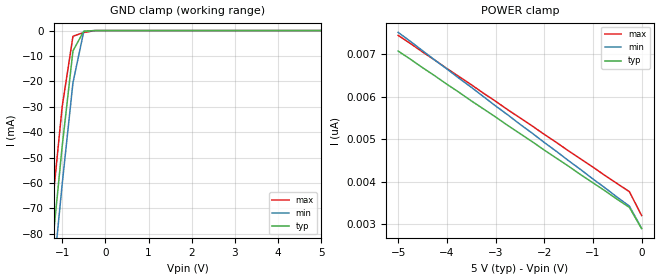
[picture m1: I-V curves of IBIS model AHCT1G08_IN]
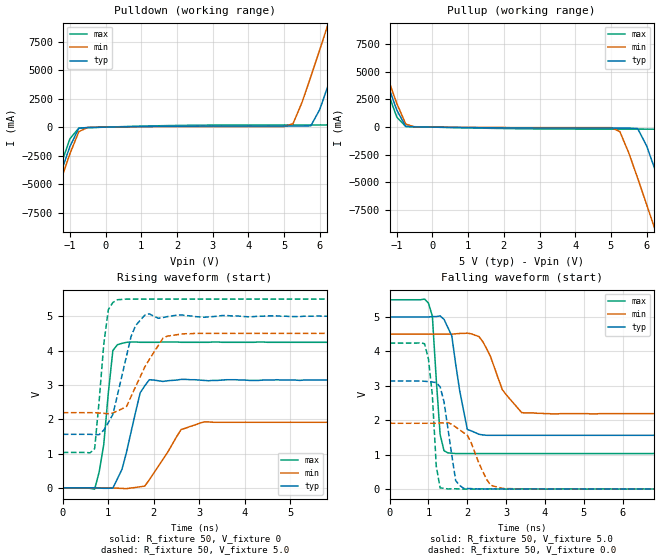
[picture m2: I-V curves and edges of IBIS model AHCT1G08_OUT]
| TEXAS INSTRUMENTS INCORPORATED
| Standard Linear and Logic Group
| IBIS Model of SN74AHCT1G08
| SINGLE 2-INPUT POSITIVE-AND GATE
| SOT 5-pin (DCK) and SOT 5-pin (DBV) Package
[IBIS Ver]   3.2
[Comment Char]  |_char
[File Name]   ahct1g08.ibs
[File Rev]   2.0 J_die
[Date]   May 24, 2000
[Source]   Data created from HSPICE simulations at TI-SLL.
[Notes]   The following is an IBIS list for the AHCT1G08.
|   Please contact sllibis@ti.com with questions and
|   comments concerning SLL IBIS models.
[Disclaimer] Property of Texas Instruments Incorporated.  Unauthorized
   reproduction and/or distribution is strictly prohibited.
   This product is protected under copyright law.
   Created 2000, (C) Copyright 2000, Texas Instruments Inc.,
   All Rights Reserved.
   UNLESS THERE IS A SIGNED, WRITTEN AGREEMENT TO THE
   CONTRARY, TEXAS INSTRUMENTS () IS PROVIDING THE IBIS
   MODELS  AND WITHOUT ANY WARRANTY, EXPRESSED OR
   IMPLIED.  TI assumes no liability for:
   1) the accuracy of the IBIS models provided to your
   company;
   2) the proper functioning of these IBIS Models in your
   design or for any resulting applications; or
   3) infringement of patents, copyrights or intellectual
   property rights resulting from your use of these IBIS
   models.
   TI provides IBIS Models as a service to our customers.
   You and your company shall not distribute, sell or give
   these models to anyone else without prior written
   permission from TI.
   TI reserves the right to make changes to our products or
   to discontinue any semiconductor product or service
   without notice, and advises our customers to obtain the
   latest version of relevant information to verify, before
   placing orders, that the information being relied on is
   current.
   Please be aware that your receipt and use of the IBIS
   information provided shall serve as acceptance of these
   terms and conditions.  If you do not accept these terms,
   you should return or destroy the IBIS models and any
   other accompanying information immediately.
|   Component AHCT1G08_DCK
[Component]   AHCT1G08_DCK
[Manufacturer]  Texas Instruments, Inc.
[Package]
|   typ   min   max
R_pkg   0.020   0.017   0.025
L_pkg   0.998nH   0.881nH   1.069nH
C_pkg   0.146pF   0.118pF   0.205pF
[Pin]   signal_name   model_name   R_pin   L_pin   C_pin
1   A   AHCT1G08_IN   0.019   1.069nH   0.162pF
2   B   AHCT1G08_IN   0.018   0.881nH   0.121pF
3   GND   GND   0.017   1.031nH   0.205pF
4   Y   AHCT1G08_OUT   0.020   0.960nH   0.124pF
5   VCC   POWER   0.025   1.049nH   0.118pF
|   Component AHCT1G08_DBV
[Component]   AHCT1G08_DBV
[Manufacturer]  Texas Instruments, Inc.
[Package]
|   typ   min   max
R_pkg   0.025   0.021   0.029
L_pkg   1.529nH   1.312nH   1.906nH
C_pkg   0.156pF   0.110pF   0.240pF
[Pin]   signal_name   model_name   R_pin   L_pin   C_pin
1   A   AHCT1G08_IN   0.021   1.511nH   0.144pF
2   B   AHCT1G08_IN   0.023   1.312nH   0.138pF
3   GND   GND   0.029   1.906nH   0.240pF
4   Y   AHCT1G08_OUT   0.026   1.541nH   0.150pF
5   VCC   POWER   0.025   1.374nH   0.110pF
| Models and submodels in the file (2): AHCT1G08_IN (Input), AHCT1G08_OUT (Output)
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|   Model AHCT1G08_IN
[Model]   AHCT1G08_IN
Model_type  Input
Polarity   Inverting
Vinl = 0.8
Vinh = 2.0
| variable   typ   min   max
C_comp   1.24pf   0.93pf   1.55pf
[Temperature Range]   25   85   -40
[Voltage Range]   5.0   4.5   5.5
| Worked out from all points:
|   GND clamp passes 1 mA (typ) near -0.52 V on its own axis
[GND Clamp]
|   Voltage   I(typ)   I(min)   I(max)
-5V       -773mA     -786mA     -758mA
-1.5V     -133mA     -148mA     -117mA
-1.25V    -88.7mA    -104mA     -72.7mA
-1V       -45.6mA    -60.5mA    -30mA
-750mV    -7.99mA    -20.5mA    -2.23mA
-500mV    -233uA     -353uA     -759uA
-250mV    -2.63nA    -182nA     -26.9uA
5V        2.9nA      3.64nA     2.54nA
[POWER Clamp]
|   Voltage   I(typ)   I(min)   I(max)
-5V       7.08nA     7.52nA     7.45nA
-1.5V     4.37nA     4.5nA      4.73nA
-250mV    3.4nA      3.43nA     3.77nA
0V        2.9nA      2.91nA     3.21nA
|   Model AHCT1G08_OUT
[Model]   AHCT1G08_OUT
Model_type  Output
Polarity   Inverting
Vmeas = 2.50v
Cref = 15pf
| variable   typ   min   max
C_comp   3.12pf   2.34pf   3.90pf
[Temperature Range]   25   85   -40
[Voltage Range]   5.0   4.5   5.5
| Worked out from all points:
|   slope of the pulldown table from 0 to 0.75 V, typ, clamps not added: 18.8 ohm
|   slope of the pullup table from 0 to 0.75 V, typ, clamps not added: 25.3 ohm
|   rising waveform, R_fixture 50, V_fixture 0: 20-80 % time 336ps typ, 543ps min, 203ps max; typ from 0 V to 3.14 V
|   falling waveform, R_fixture 50, V_fixture 5.0: 20-80 % time 292ps typ, 554ps min, 156ps max; typ from 5 V to 1.56 V
|   rising waveform, R_fixture 50, V_fixture 5.0: 20-80 % time 364ps typ, 547ps min, 187ps max; typ from 1.56 V to 5 V
|   falling waveform, R_fixture 50, V_fixture 0.0: 20-80 % time 246ps typ, 438ps min, 155ps max; typ from 3.14 V to 0 V
[Pulldown]
|   Voltage   I(typ)   I(min)   I(max)
-5V       -40.9A     -41.4A     -40.3A
-1.75V    -8.76A     -9.39A     -8.09A
-1V       -1.69A     -2.33A     -1.02A
-750mV    -95.5mA    -395mA     -80.6mA
5.25V     93.4mA     298mA      192mA
5.75V     116mA      4.42A      192mA
6.25V     3.8A       9.19A      193mA
6.5V      6.17A      11.6A      931mA
6.75V     8.59A      14.1A      3.15A
7.25V     13.5A      19A        7.96A
7.5V      15.9A      21.4A      10.4A
10V       40.7A      46.2A      35.2A
[Pullup]
|   Voltage   I(typ)   I(min)   I(max)
-5V       40.7A      41.2A      40.1A
-2V       11A        11.6A      10.4A
-1.75V    8.59A      9.19A      7.96A
-1V       1.54A      2.14A      907mA
-750mV    63.6mA     284mA      62.5mA
5.25V     -84.4mA    -401mA     -178mA
5.75V     -130mA     -4.62A     -178mA
6.25V     -3.97A     -9.39A     -187mA
6.75V     -8.76A     -14.3A     -3.28A
7.25V     -13.6A     -19.2A     -8.09A
7.5V      -16.1A     -21.6A     -10.5A
10V       -40.9A     -46.4A     -35.3A
[Ramp]
| variable   typ   min   max
dV/dt_r   1.89E+00/3.19E-10   1.16E+00/5.23E-10   2.55E+00/2.03E-10
dV/dt_f   2.10E+00/2.70E-10   1.41E+00/5.15E-10   2.70E+00/1.43E-10
R_load = 50
[Rising Waveform]
R_fixture = 50
V_fixture = 0
|   Time   V(typ)   V(min)   V(max)
0s        0V         0V         0V
700ps     2.67mV     667uV      -38.7mV
900ps     -13.4mV    2.41mV     1.26V
1.1ns     -6.87mV    -3.39mV    4V
1.4ns     1.04V      -23.7mV    4.24V
1.7ns     2.77V      31.1mV     4.24V
1.9ns     3.15V      232mV      4.24V
2.6ns     3.16V      1.7V       4.24V
3.1ns     3.13V      1.92V      4.24V
25ns      3.14V      1.91V      4.24V
[Falling Waveform]
R_fixture = 50
V_fixture = 5.0
V_fixture_min = 4.5
V_fixture_max = 5.5
|   Time   V(typ)   V(min)   V(max)
0s        5V         4.5V       5.5V
1ns       5V         4.5V       5.4V
1.1ns     5.01V      4.5V       5.02V
1.3ns     5.03V      4.5V       1.58V
1.5ns     4.69V      4.5V       1.05V
2ns       1.73V      4.53V      1.03V
2.4ns     1.57V      4.28V      1.03V
2.9ns     1.56V      2.89V      1.03V
3.5ns     1.56V      2.21V      1.03V
25ns      1.56V      2.19V      1.03V
[Rising Waveform]
R_fixture = 50
V_fixture = 5.0
V_fixture_min = 4.5
V_fixture_max = 5.5
|   Time   V(typ)   V(min)   V(max)
0s        1.56V      2.19V      1.03V
700ps     1.55V      2.19V      1.14V
900ps     1.68V      2.17V      4.18V
1ns       1.9V       2.16V      5.19V
1.2ns     2.7V       2.24V      5.48V
1.5ns     4.41V      2.66V      5.5V
1.9ns     5.07V      3.74V      5.5V
2.2ns     4.96V      4.36V      5.5V
2.9ns     4.99V      4.5V       5.5V
25ns      5V         4.5V       5.5V
[Falling Waveform]
R_fixture = 50
V_fixture = 0.0
|   Time   V(typ)   V(min)   V(max)
0s        3.14V      1.91V      4.24V
900ps     3.13V      1.91V      4.22V
1ns       3.12V      1.91V      3.77V
1.1ns     3.11V      1.91V      2.72V
1.2ns     3.09V      1.91V      664mV
1.3ns     2.97V      1.92V      30.4mV
1.7ns     244mV      1.8V       5.72mV
1.9ns     22.5mV     1.64V      -1.81mV
2.9ns     2.02mV     17.5mV     -2.28mV
25ns      0V         0V         0V
